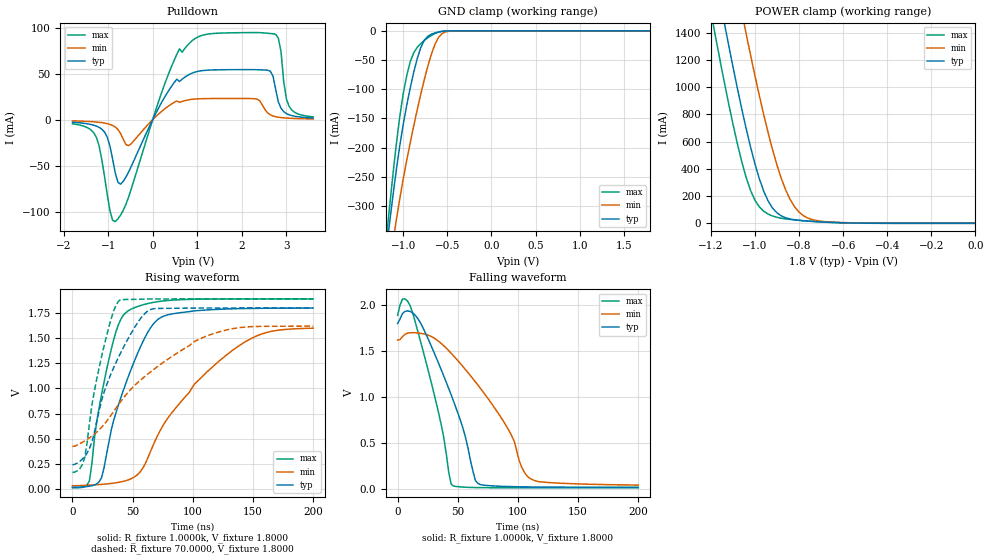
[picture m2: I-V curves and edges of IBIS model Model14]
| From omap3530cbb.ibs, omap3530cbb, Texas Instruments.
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| Model based on original model for BQ0246S_7LM
|   Sub model BQ0246S_7LM_I2C_1
[model]   Model14
|[Input Load]
|[Output Drive] LOWC
|Voltage   1.8000V
|Mode   I/O_OPEN_DRAIN
Model_type   I/O_open_drain
Polarity   Non-Inverting
Enable   Active-Low
Vinl =   0.6615V
Vinh =   1.0530V
Vmeas =   0.9000V
Cref =  15.0000pF
Rref =  70.0000
Vref =  1.8000V
C_comp   27.0699pF   15.4565pF   39.2456pF
[Temperature Range]   25.0000   0.1250k   -40.0000
[Voltage Range]   1.8000V   1.6200V   1.8900V
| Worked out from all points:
|   slope of the pulldown table from 0 to 0.27 V, typ, clamps not added: 11 ohm
|   GND clamp passes 1 mA (typ) near -0.56 V on its own axis
|   POWER clamp passes 1 mA (typ) near -0.50 V on its own axis
|   rising waveform, R_fixture 1.0000k, V_fixture 1.8000: 20-80 % time 28.9ns typ, 59.3ns min, 17.7ns max; typ from 0.018 V to 1.8 V
|   rising waveform, R_fixture 70.0000, V_fixture 1.8000: 20-80 % time 28ns typ, 63.1ns min, 16.2ns max; typ from 0.24 V to 1.8 V
|   falling waveform, R_fixture 1.0000k, V_fixture 1.8000: 20-80 % time 28ns typ, 44.1ns min, 19.5ns max; typ from 1.8 V to 0.018 V
[Pulldown]
-1.8V     -2.87mA    -1.375mA   -4.529mA
-1.26V    -7.103mA   -2.596mA   -19.64mA
-1.02V    -19mA      -4.333mA   -81.54mA
-840mV    -58mA      -8.066mA   -110.9mA
-540mV    -56.9mA    -28.26mA   -84.16mA
540mV     44.06mA    20.37mA    70.88mA
1.02V     52.59mA    22.64mA    90.07mA
2.34V     54.31mA    22.37mA    94.71mA
2.58V     53.76mA    7.273mA    93.96mA
2.76V     32.74mA    3.19mA     92.69mA
3.06V     5.312mA    1.538mA    14.56mA
3.6V      1.833mA    776uA      3.052mA
[GND_clamp]
-1.8V     -1.221A    -1.151A    -1.363A
-1.2V     -386.5mA   -449.7mA   -370.2mA
-1.16V    -335.5mA   -406.8mA   -309.4mA
-1.08V    -240.2mA   -325.8mA   -196.3mA
-1V       -160.3mA   -253.8mA   -107.7mA
-960mV    -127.1mA   -221.5mA   -76.33mA
-920mV    -97.28mA   -191.1mA   -52.71mA
-840mV    -46.78mA   -134.3mA   -27.94mA
-720mV    -9.253mA   -59.82mA   -11.79mA
-600mV    -1.888mA   -11.35mA   -2.27mA
-480mV    -137.6uA   -650.4uA   -84.11uA
1.8V      510.5nA    3.198uA    487.6nA
[POWER_clamp]
-1.8V     7.644A     8.363A     7.23A
-1.2V     2.004A     2.755A     1.56A
-1.18V    1.829A     2.578A     1.386A
-1.14V    1.486A     2.23A      1.05A
-1.12V    1.32A      2.059A     889mA
-1.04V    700.2mA    1.398A     339.6mA
-1V       439.3mA    1.088A     170.8mA
-940mV    164.6mA    666.7mA    68.12mA
-860mV    40.26mA    244.2mA    32.16mA
-820mV    25.74mA    121.5mA    25.05mA
-760mV    16.31mA    38.76mA    16.75mA
0V        510.5nA    462.5nA    537.3nA
[Ramp]
dV/dt_r   0.2712m/26.3758n   0.8307m/47.8314n   0.3415m/16.4633n
dV/dt_f   1.0688/27.7327n   0.9465/45.1789n   1.1265/19.2750n
R_load = 1.0000k
[Rising Waveform]
R_fixture = 1.0000k
V_fixture = 1.8000
V_fixture_min = 1.6200
V_fixture_max = 1.8900
0s        17.75mV    32.74mV    11.97mV
14.14ns   28.2mV     38.7mV     83mV
24.24ns   115.1mV    46.27mV    943.3mV
36.36ns   767mV      62.35mV    1.573V
46.46ns   1.119V     91.37mV    1.773V
62.63ns   1.559V     310.1mV    1.844V
76.77ns   1.723V     660.6mV    1.871V
103ns     1.772V     1.061V     1.887V
141.4ns   1.793V     1.447V     1.889V
200ns     1.799V     1.599V     1.889V
[Rising Waveform]
R_fixture = 70.0000
V_fixture = 1.8000
V_fixture_min = 1.6200
V_fixture_max = 1.8900
0s        240mV      423.8mV    164mV
10.1ns    321.9mV    477.9mV    309.4mV
16.16ns   468.7mV    526.6mV    837.9mV
22.22ns   784.1mV    589.4mV    1.21V
32.32ns   1.154V     738.3mV    1.698V
38.38ns   1.313V     842.2mV    1.87V
56.57ns   1.695V     1.083V     1.887V
66.67ns   1.79V      1.181V     1.889V
123.2ns   1.799V     1.566V     1.89V
200ns     1.8V       1.619V     1.89V
[Falling Waveform]
R_fixture = 1.0000k
V_fixture = 1.8000
V_fixture_min = 1.6200
V_fixture_max = 1.8900
0s        1.8V       1.619V     1.889V
4.04ns    1.908V     1.657V     2.066V
12.12ns   1.919V     1.7V       1.929V
32.32ns   1.421V     1.624V     924.1mV
46.46ns   954.7mV    1.448V     31.37mV
64.65ns   92.37mV    1.165V     15.39mV
68.69ns   47.47mV    1.096V     14.54mV
92.93ns   26.01mV    626.2mV    12.62mV
109.1ns   21.92mV    122.9mV    12.25mV
200ns     18.14mV    42.12mV    11.98mV
